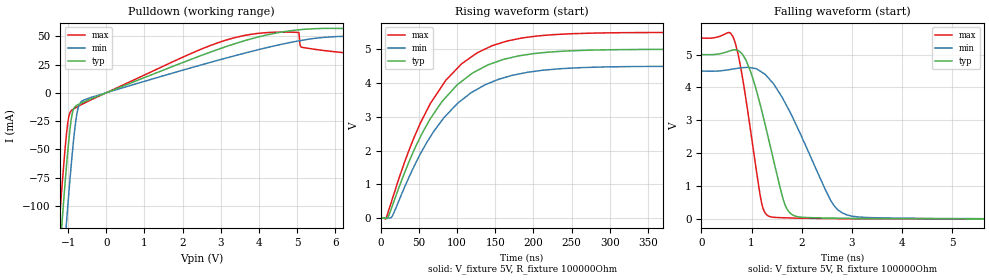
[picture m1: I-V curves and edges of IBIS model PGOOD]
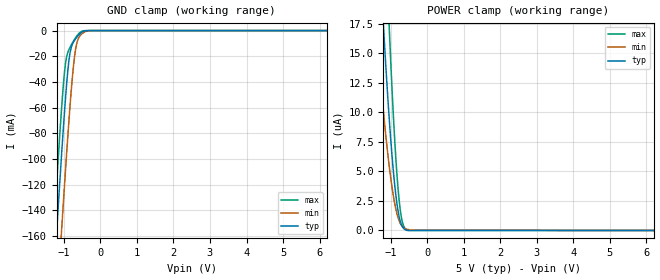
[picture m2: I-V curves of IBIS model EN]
|Texas Instruments Incorporated
| Single phase DCAP and D-CAP2 Controller
| Marketing part#   Digital Voltage Range   Package-type   #pins
| TPS51518RUKR   4.5V - 5.5V   QFN   20
| TPS51518RUKR   4.5V - 5.5V   QFN   20
[IBIS Ver]   4.1
[File name]   tps51518.ibs
[File Rev]   1.0
[Date]   6/28/2012
[Source]
| Texas Instruments Incorporated.
| Analog-eLab Design Center, HPA
| 12500 TI Blvd
| Dallas, TX -75243
| e-mail: elab_scm_ibis@list.ti.com
[Notes]   Revision History:
| Rev 1.0: 6/28/2012
| - Initial version of the model
| - Model generated from simulations in TISPICE
| - C_comp although listed in numerical order of value are
|   obtained from varying PVT conditions. For PVT conditions for
|   each specific value refer the buffer description under
|   respective [Model]. IBIS model user is responsible for using
|   appropriate C_comp to simulate for Signal Integrity.
|  - Combined Non-monotonicity warnings of pulldown for PGOOD are minor
|   and reflect SPICE transistor simulations and can be ignored.
[Disclaimer]
| This model is designed as an aid for customers of Texas Instruments.
| TI and its licensors and suppliers make no warranties, either expressed
| or implied, with respect to this  model, including the warranties of
| merchantability or fitness for a particular purpose. The model is
| provided solely on an "as is" basis. The entire risk as to its quality
| and performance is with the customer.
[Copyright]
 (C) Copyright 2012 Texas Instruments Incorporated.All rights reserved.
|   TPS51518
[Component]   TPS51518
[Manufacturer]   TI
[Package]
|   typ   min   max
R_pkg   0.1   0.08   0.12
L_pkg   1.0nH   0.8nH   1.2nH
C_pkg   0.4pF   0.32pF   0.48pF
[Pin]  signal_name   model_name   R_pin   L_pin   C_pin
1   GSNS   NC   NA   NA   NA
2   V3   NC   NA   NA   NA
3   V2   NC   NA   NA   NA
4   V1   NC   NA   NA   NA
5   V0   NC   NA   NA   NA
6   VREF   NC   NA   NA   NA
7   PGOOD   PGOOD   NA   NA   NA
8   VID0   NC   NA   NA   NA
9   VID1   NC   NA   NA   NA
10   EN   EN   NA   NA   NA
11   BST   NC   NA   NA   NA
12   SW   NC   NA   NA   NA
13   DRVH   NC   NA   NA   NA
14   DRVL   NC   NA   NA   NA
15   V5IN   POWER   NA   NA   NA
16   MODE   NC   NA   NA   NA
17   GND   GND   NA   NA   NA
18   TRIP   NC   NA   NA   NA
19   SLEW   NC   NA   NA   NA
20   VSNS   NC   NA   NA   NA
| Models and submodels in the file (2): PGOOD (Open_drain), EN (Input)
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|   PGOOD Model
[Model]   PGOOD
Model_type   Open_drain
Polarity   Non-Inverting
Vmeas = 2.5
Vref = 5
Cref = 1pF
Rref = 100000
|   typ   min   max
C_comp   1pF   1pF   1pF
[Voltage Range]   5   4.5   5.5
[Temperature Range]   27   125   -40
[Pullup Reference]   5   4.5   5.5
[Pulldown Reference]   -0   -0   -0
[Power Clamp Reference]   5   4.5   5.5
[GND Clamp Reference]   -0   -0   -0
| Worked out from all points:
|   slope of the pulldown table from 0 to 0.75 V, typ, clamps not added: 74.5 ohm
|   falling waveform, V_fixture 5V, R_fixture 100000Ohm: 20-80 % time 482ps typ, 825ps min, 326ps max; typ from 5 V to 0.004 V
|   rising waveform, V_fixture 5V, R_fixture 100000Ohm: 20-80 % time 77.7ns typ, 80.9ns min, 75.9ns max; typ from 0.004 V to 5 V
[Pulldown]
|   Voltage   I(typ)   I(min)   I(max)
-5V       -1.997A    -2.043A    -1.969A
-1.25V    -155.9mA   -208mA     -123.3mA
-1.16V    -115.3mA   -167mA     -83.1mA
-1.04V    -64.26mA   -114mA     -35.76mA
-980mV    -41.77mA   -88.73mA   -20.77mA
-800mV    -11.76mA   -25.37mA   -13.24mA
-650mV    -9.078mA   -7.66mA    -10.44mA
3.16V     41.06mA    30.88mA    46.8mA
5.05V     55.7mA     45.94mA    53.36mA
6.31V     56.79mA    50.03mA    35.21mA
6.4V      42.64mA    50.1mA     34.94mA
9.97V     32.99mA    50.8mA     28.32mA
[Ramp]
R_load = 100000
|   typ   min   max
dV/dt_r   2.99809/7.77413e-08   2.6961/8.09044e-08   3.29815/7.59114e-08
dV/dt_f   2.99773/4.82394e-10   2.69589/8.24581e-10   3.29789/3.25716e-10
[Falling Waveform]
V_fixture = 5V
V_fixture_min = 4.5V
V_fixture_max = 5.5V
R_fixture = 100000Ohm
C_fixture = 0F
|   Time   V(typ)   V(min)   V(max)
0s        5V         4.498V     5.5V
675.8ps   5.14V      4.571V     5.352V
892.6ps   4.82V      4.608V     3.6V
1.17ns    3.497V     4.498V     741mV
1.274ns   2.861V     4.395V     182.9mV
1.71ns    300.9mV    3.417V     39.74mV
2.649ns   29.86mV    405.8mV    16.66mV
3.252ns   19.6mV     54.34mV    11.69mV
9.156ns   4.97mV     7.271mV    3.627mV
500ns     3.704mV    4.379mV    3.509mV
[Rising Waveform]
V_fixture = 5V
V_fixture_min = 4.5V
V_fixture_max = 5.5V
R_fixture = 100000Ohm
C_fixture = 0F
|   Time   V(typ)   V(min)   V(max)
0s        3.704mV    4.379mV    3.509mV
6.573ns   -6.917mV   -558.8uV   -13.2mV
14.4ns    328.3mV    38.82mV    527.1mV
42.37ns   1.958V     1.481V     2.33V
64.87ns   2.948V     2.41V      3.397V
85.27ns   3.583V     3.038V     4.087V
126.1ns   4.37V      3.816V     4.895V
171.7ns   4.76V      4.227V     5.276V
236.7ns   4.942V     4.428V     5.448V
500ns     5.001V     4.498V     5.5V
|   EN Model
[Model]   EN
Model_type   Input
Vinl = 0.8
Vinh = 3.5
|   typ   min   max
C_comp   1pF   1pF   1pF
[Voltage Range]   5   4.5   5.5
[Temperature Range]   27   125   -40
[Power Clamp Reference]   5   4.5   5.5
[GND Clamp Reference]   -0   -0   -0
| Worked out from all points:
|   GND clamp passes 1 mA (typ) near -0.49 V on its own axis
[GND Clamp]
|   Voltage   I(typ)   I(min)   I(max)
-5V       -2.024A    -2.079A    -1.99A
-1.43V    -266.3mA   -326.7mA   -228.1mA
-1.25V    -181.6mA   -242.1mA   -143.5mA
-1.19V    -154mA     -214.3mA   -116mA
-1.07V    -100.3mA   -159.6mA   -64.04mA
-950mV    -51.22mA   -107mA     -24.67mA
-830mV    -17.25mA   -58.53mA   -13.07mA
-740mV    -9.141mA   -28.57mA   -8.413mA
-680mV    -6.512mA   -14.82mA   -5.686mA
-590mV    -3.363mA   -5.505mA   -2.343mA
-470mV    -681.9uA   -1.712mA   -195uA
9.97V     0A         0A         0A
[POWER Clamp]
|   Voltage   I(typ)   I(min)   I(max)
-5V       79.82uA    79.73uA    88.41uA
-1.4V     28.62uA    17.33uA    37.27uA
-1.37V    27.06uA    16.16uA    36.66uA
-1.19V    16.87uA    9.771uA    28.86uA
-1.04V    9.433uA    5.433uA    17.17uA
-920mV    4.765uA    2.794uA    9.294uA
-860mV    2.994uA    1.818uA    6.113uA
-800mV    1.669uA    1.093uA    3.571uA
-710mV    519.2nA    442.7nA    1.149uA
-650mV    187nA      231.7nA    405.2nA
-590mV    45.95nA    126.8nA    105nA
9.97V     0A         0A         0A
